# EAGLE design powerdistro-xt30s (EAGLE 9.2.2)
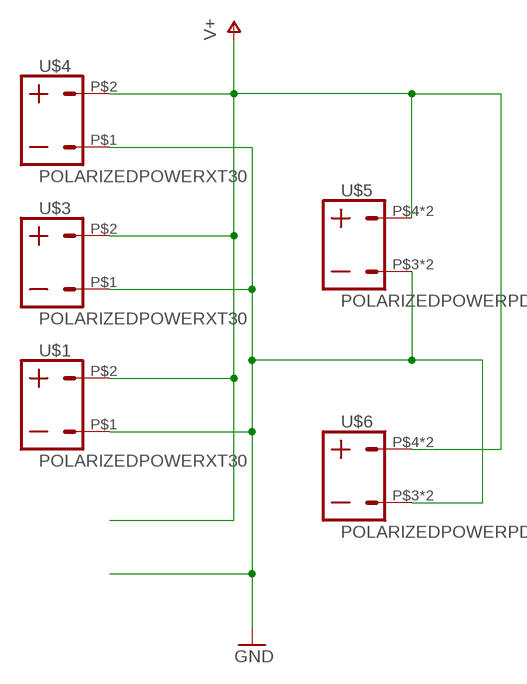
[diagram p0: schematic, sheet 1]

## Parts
U$1  POLARIZEDPOWERXT30  [XT30]
U$3  POLARIZEDPOWERXT30  [XT30]
U$4  POLARIZEDPOWERXT30  [XT30]
U$5  POLARIZEDPOWERPDB  [PDBCONN]
U$6  POLARIZEDPOWERPDB  [PDBCONN]

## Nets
GND: U$1.P$1 U$3.P$1 U$4.P$1 U$5.P$3 U$5.P$6 U$6.P$3 U$6.P$6
V+: U$1.P$2 U$3.P$2 U$4.P$2 U$5.P$4 U$5.P$5 U$6.P$4 U$6.P$5

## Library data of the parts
U$1 U$3-U$6 = connector:POLARIZEDPOWER

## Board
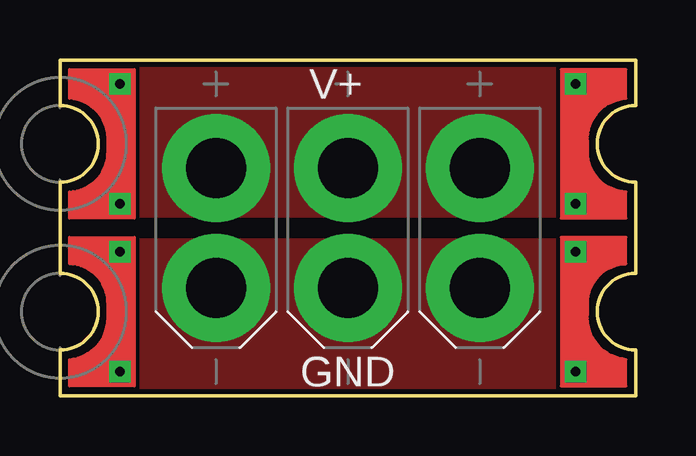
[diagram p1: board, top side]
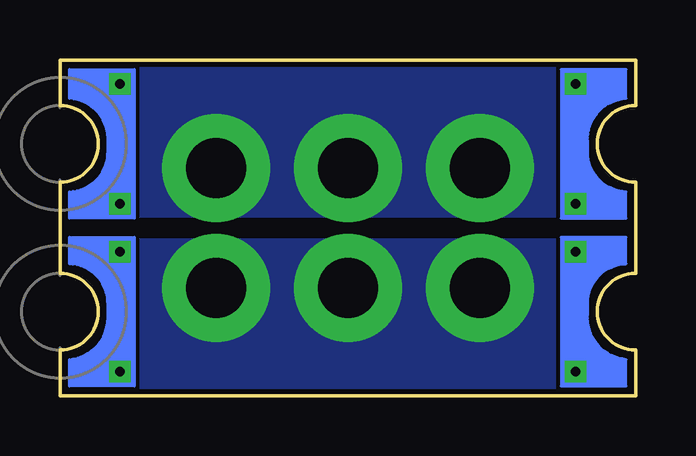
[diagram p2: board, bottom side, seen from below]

Size 24 x 14 mm. Coordinates in mm from the lower left corner, seen from the top.
Outline: 0,5.1 0,8.9 arc90 1.6,10.5 arc90 0,12.1 0,14 24,14 24,12.1 arc90 22.4,10.5 arc90 24,8.9 24,5.1 arc90 22.4,3.5 arc90 24,1.9 24,0 0,0 0,1.9 arc90 1.6,3.5 arc90 0,5.1
Copper layers (1*16): Top 0.035mm / dielectric 1.5mm / Bottom 0.035mm
Design rules "default *": minimum track width 6mil, minimum drill 0.35mm, track to track 6mil, track to pad 6mil, pad to pad 6mil, via to via 6mil, smd to smd 6mil, copper to edge 8mil, drill to drill 6mil, minimum pad ring 10mil, minimum via ring 8mil, stop-mask expansion 4mil, vias tented up to drill 0mil, thermal gap 10mil

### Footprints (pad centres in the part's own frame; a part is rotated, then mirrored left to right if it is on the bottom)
XT30 = drill 2.5 pad 4.5: P$1 2.5,0; P$2 -2.5,0
PDBCONN = drill 0.4 square: P$3 2.5,2.5; P$4 2.5,4.5; P$5 2.5,9.5; P$6 2.5,-2.5

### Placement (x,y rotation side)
U$1  6.5,7 270 top
U$3  12,7 270 top
U$4  17.5,7 270 top
U$5  0,3.5 0 top
U$6  24,3.5 0 bottom

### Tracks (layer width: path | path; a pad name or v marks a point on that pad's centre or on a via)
GND
  pour Top: -1,6.5 26.5,6.5 26.5,-0.5 -1,-0.5
  pour Bottom: -1.5,6.5 27,6.5 27,-1 -1.5,-1
V+
  pour Top: -1,7.5 26.5,7.5 26.5,15 -1,15
  pour Bottom: -1.5,7.5 27,7.5 27,15.5 -1.5,15.5

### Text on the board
tPlace: V+ | GND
